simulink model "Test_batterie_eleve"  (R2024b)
settings: Solver=VariableStepAuto  StartTime=0.0  StopTime=288000  RelTol=1e-3
libraries: fl_lib x7, nesl_utility x6, ee_lib x4, simulink x2, batteryecm_lib x1, simulink_extras x1

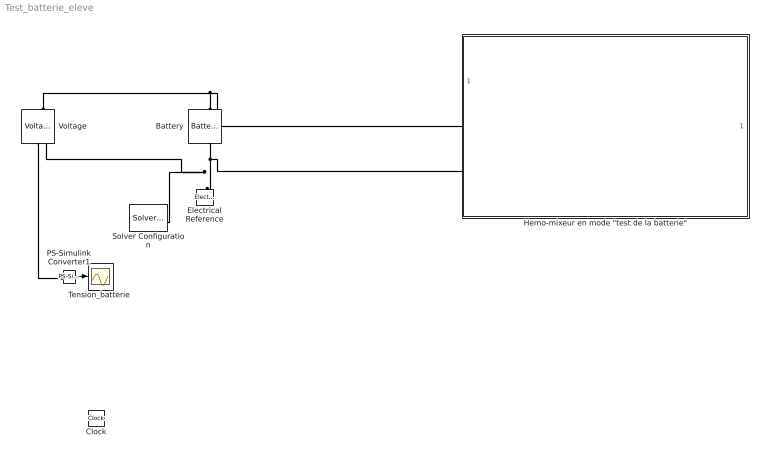
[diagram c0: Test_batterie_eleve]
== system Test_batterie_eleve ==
  Battery : batteryecm_lib/Battery  Vnom=9 V  prm_dir=simscape.enum.battery.prm_dir.disabled  R1_dis=2 Ohm  R1_ch=2 Ohm  R1=0.2 Ohm  prm_AH=2  AH=5 Ah  V1=10.8 V  AH1=0.76 Ah  prm_R2=1  R2=2000 Ohm  Tmeas=298.15 K  charge_measurement_port=simscape.enum.battery.enable.no  prm_dyn=1  Rp1=0.005 Ohm  tau1=30 s  Rp2=0.005 Ohm  tau2=30 s  Rp3=0.005 Ohm  tau3=30 s  Rp4=0.005 Ohm  tau4=30 s  Rp5=0.005 Ohm  tau5=30 s  prm_fade=1  N_fade=100  AH_fade=45 hr*A  R1_fade=2.02 Ohm  R1_ch_fade=2.02 Ohm  V1_fade=10.35 V  prm_age=simscape.enum.battery.prm_age.disabled  prm_age_OCV=simscape.enum.battery.prm_age_OCV.OCV  OCV_age=0.9  SOC_age=60  Tmeas_age=298.15 K  delta_time_age_vec=[0] d  temperature_age_vec=[273] K  OCV_scaling_age=2.2134e6  OCV_offset_age=1.632e6  temp_exp_age=0.515833569 V  t_exp_age=0.75  Vnom_T2=12 V  R1_T2=2.2 Ohm  R1_T2_dis=2.2 Ohm  R1_T2_ch=2.2 Ohm  V1_T2=11.4 V  R2_T2=2200 Ohm  Rp1_T2=0.005 Ohm  tau1_T2=30 s  Rp2_T2=0.005 Ohm  tau2_T2=30 s  Rp3_T2=0.005 Ohm  tau3_T2=30 s  Rp4_T2=0.005 Ohm  tau4_T2=30 s  Rp5_T2=0.005 Ohm  tau5_T2=30 s  Tmeas2=273.15 K  thermal_port=simscape.enum.thermaleffects.omit  thermal_mass=30000 J/K  i_specify=off  i_priority=None  i=0 A  i_nominal_specify=off  i_nominal_value=1  i_nominal_unit=A  v_specify=off  v_priority=None  v=14 V  v_nominal_specify=off  v_nominal_value=1  v_nominal_unit=V  charge_specify=on  charge_priority=High  charge=3.8 hr*A  charge_nominal_specify=off  charge_nominal_value=1  charge_nominal_unit=hr*A  num_cycles_specify=off  num_cycles_priority=High  num_cycles=0  num_cycles_nominal_specify=off  num_cycles_nominal_value=1  num_cycles_nominal_unit=1  temperature_specify=off  temperature_priority=High  temperature=298.15 K  temperature_nominal_specify=off  temperature_nominal_value=1  temperature_nominal_unit=K
  Electrical Reference : fl_lib/Electrical/Electrical Elements/Electrical Reference
  "Hemo-mixeur en mode \"test de la batterie\"" : Subsystem
  PS-Simulink Converter1 : nesl_utility/PS-Simulink Converter  PhysicalDomain=network_engine_domain  SubClassName=ps_output  LeftPortType=input  RightPortType=output  PseudoPeriodic=off  Frequencies=[]  VectorFormat=1-D array  Unit=inherit  AffineConversion=off
  Solver Configuration : nesl_utility/Solver Configuration  PhysicalDomain=network_engine_domain  SubClassName=solver  LeftPortType=input  RightPortType=generic  Tones=[]  Harmonics=[]  SimulateNoise=off  Profile=off  UseLocalSampling=off  EnableSwitchedLinearOptims=on  FrequencyDomain=off  UseCCode=off  RelTol=0.001  AbsTol=1e-06  MinStep=1e-09  ToWorkspace=off  RevertToSquareIcSolve=off  NumHomotopyIterations=100  PhasorMode=off  PhasorModeNumHarmonics=1  ConsistencySolver=NEWTON_FTOL  IndexReductionMethod=DerivativeReplacement  DoDC=off  ResidualTolerance=1e-09  ConsistencyTolSource=GLOBAL  ConsistencyAbsTol=0.001  ConsistencyRelTol=0.001  ConsistencyTolFactor=0.001  UseLocalSolver=off  LocalSolverChoice=NE_BACKWARD_EULER_ADVANCER  ResolveIndetEquations=on  FunctionEvalNumThread=1  LocalSolverSampleTime=0.001  DoFixedCost=off  MaxNonlinIter=3  MaxModeIter=2  ComputeImpulses=off  ImpulseIterations=2  LinearAlgebra=auto  LinearAlgebraNumThread=0  EquationFormulation=NE_TIME_EF  DelaysMemoryBudget=1024  AutomaticFiltering=on  FilteringTimeConstant=0.001  PartitionStorageMethod=AS_NEEDED  PartitionMemoryBudget=1024  PartitionMethod=ROBUST  MultibodyUseLocalSolver=off  MultibodyLocalSolverChoice=ODE1  MultibodyLocalSolverSampleTime=0.001
  "Tension_batterie " : Scope
  Voltage : fl_lib/Electrical/Electrical Sensors/Voltage Sensor
  Clock : Clock
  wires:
  PS-Simulink Converter1/1 -> "Tension_batterie "/1
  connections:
  Voltage/RConn1 -- PS-Simulink Converter1/LConn1
  Voltage/LConn1 -- "Hemo-mixeur en mode \"test de la batterie\""/LConn1 -- Battery/LConn1
  Battery/RConn1 -- Solver Configuration/RConn1 -- Voltage/RConn2 -- "Hemo-mixeur en mode \"test de la batterie\""/LConn2 -- Electrical Reference/LConn1

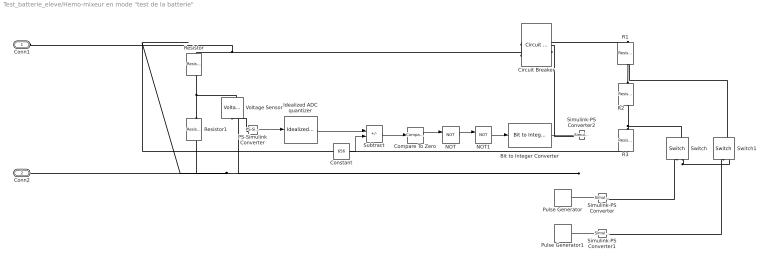
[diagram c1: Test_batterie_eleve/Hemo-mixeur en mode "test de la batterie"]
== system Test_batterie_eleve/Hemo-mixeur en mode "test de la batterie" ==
  Bit to Integer Converter : simulink/Logic and Bit Operations/Bit to Integer Converter  nbits=1  bitOrder=MSB first  signedOutputValues=Unsigned  outDtype=double  outDtypeSigned=Inherit via internal rule
  Circuit Breaker : ee_lib/Switches & Breakers/Circuit Breaker  R_closed=0.001 Ohm  G_open=1e-6 1/Ohm  threshold=0.5 V  breaker_behavior=ee.enum.switches.breakerBehavior.zeroCrossingDisable
  Compare To Zero : simulink/Logic and Bit Operations/Compare To Zero  relop=<=  OutDataTypeStr=boolean  ZeroCross=off
  Constant : Constant  Value=656
  Idealized ADC quantizer : simulink_extras/Additional Discrete/Idealized ADC quantizer  NumberOfConverterBits=10  Vmin=0  Vmax=5  OutputDataType=uint32  OutputNegativeValues=off
  NOT : Logic  Operator=NOT  IconShape=distinctive  AllPortsSameDT=off  OutDataTypeStr=boolean
  NOT1 : Logic  Operator=NOT  IconShape=distinctive  AllPortsSameDT=off
  PS-Simulink Converter : nesl_utility/PS-Simulink Converter  PhysicalDomain=network_engine_domain  SubClassName=ps_output  LeftPortType=input  RightPortType=output  PseudoPeriodic=off  Frequencies=[]  VectorFormat=inherit  Unit=inherit  AffineConversion=off
  Pulse Generator : DiscretePulseGenerator  PulseType=Time based  Period=120  PulseWidth=8.3  VectorParams1D=off
  Pulse Generator1 : DiscretePulseGenerator  PulseType=Time based  Period=120  PulseWidth=8.3  PhaseDelay=60  VectorParams1D=off
  R1 : ee_lib/Passive/Resistor  R=86 Ohm  enable_R_tol=1  R_tol=1  tol_distribution=1  nSigma=4  enable_operating_limits=0  operating_limit_action=2  power_rating=1 W  max_working_voltage=100 V  noise_mode=0  Tdevice=25 degC  sample_time=1e-3 s  repeatability=1  user_seed=0  auto_seed=3264415495  fault_action=simscape.enum.assert.action.none  t_fault=1 s  power_derating_T1=70 degC  power_derating_T2=155 degC  operating_temperature_range_vec=[-50, 150] degC  alpha=3.93e-3 1/K  Tmeas=25 degC  thermal_mass=100 J/K  temperature_specify=off  temperature_priority=High  temperature=298.15 K  temperature_nominal_specify=off  temperature_nominal_value=1  temperature_nominal_unit=K
  R2 : ee_lib/Passive/Resistor  R=14 Ohm  enable_R_tol=1  R_tol=1  tol_distribution=1  nSigma=4  enable_operating_limits=0  operating_limit_action=2  power_rating=1 W  max_working_voltage=100 V  noise_mode=0  Tdevice=25 degC  sample_time=1e-3 s  repeatability=1  user_seed=0  auto_seed=3467225173  fault_action=simscape.enum.assert.action.none  t_fault=1 s  power_derating_T1=70 degC  power_derating_T2=155 degC  operating_temperature_range_vec=[-50, 150] degC  alpha=3.93e-3 1/K  Tmeas=25 degC  thermal_mass=100 J/K  temperature_specify=off  temperature_priority=High  temperature=298.15 K  temperature_nominal_specify=off  temperature_nominal_value=1  temperature_nominal_unit=K
  R3 : ee_lib/Passive/Resistor  R=200 Ohm  enable_R_tol=1  R_tol=1  tol_distribution=1  nSigma=4  enable_operating_limits=0  operating_limit_action=2  power_rating=1 W  max_working_voltage=100 V  noise_mode=0  Tdevice=25 degC  sample_time=1e-3 s  repeatability=1  user_seed=0  auto_seed=4244480622  fault_action=simscape.enum.assert.action.none  t_fault=1 s  power_derating_T1=70 degC  power_derating_T2=155 degC  operating_temperature_range_vec=[-50, 150] degC  alpha=3.93e-3 1/K  Tmeas=25 degC  thermal_mass=100 J/K  temperature_specify=off  temperature_priority=High  temperature=298.15 K  temperature_nominal_specify=off  temperature_nominal_value=1  temperature_nominal_unit=K
  Resistor : fl_lib/Electrical/Electrical Elements/Resistor  R=23.7 kOhm  i_specify=off  i_priority=None  i=0 A  i_nominal_specify=off  i_nominal_value=1  i_nominal_unit=A  v_specify=off  v_priority=None  v=0 V  v_nominal_specify=off  v_nominal_value=1  v_nominal_unit=V
  Resistor1 : fl_lib/Electrical/Electrical Elements/Resistor  R=10 kOhm  i_specify=off  i_priority=None  i=0 A  i_nominal_specify=off  i_nominal_value=1  i_nominal_unit=A  v_specify=off  v_priority=None  v=0 V  v_nominal_specify=off  v_nominal_value=1  v_nominal_unit=V
  Simulink-PS Converter : nesl_utility/Simulink-PS Converter  PhysicalDomain=network_engine_domain  SubClassName=ps_input  LeftPortType=input  RightPortType=output  PseudoPeriodic=off  Frequencies=[]  NoiseDistribution=none  NoiseParameters=[]  Unit=1  AffineConversion=off  FilteringAndDerivatives=provide  SimscapeFilterOrder=1  InputFilterTimeConstant=0.001  UdotUserProvided=0
  Simulink-PS Converter1 : nesl_utility/Simulink-PS Converter  PhysicalDomain=network_engine_domain  SubClassName=ps_input  LeftPortType=input  RightPortType=output  PseudoPeriodic=off  Frequencies=[]  NoiseDistribution=none  NoiseParameters=[]  Unit=1  AffineConversion=off  FilteringAndDerivatives=provide  SimscapeFilterOrder=1  InputFilterTimeConstant=0.001  UdotUserProvided=0
  Simulink-PS Converter2 : nesl_utility/Simulink-PS Converter  PhysicalDomain=network_engine_domain  SubClassName=ps_input  LeftPortType=input  RightPortType=output  PseudoPeriodic=off  Frequencies=[]  NoiseDistribution=none  NoiseParameters=[]  Unit=1  AffineConversion=off  FilteringAndDerivatives=provide  SimscapeFilterOrder=1  InputFilterTimeConstant=0.001  UdotUserProvided=0
  Subtract : Sum  Inputs=+-
  Switch : fl_lib/Electrical/Electrical Elements/Switch  R_closed=0.01 Ohm  G_open=1e-8 1/Ohm  Threshold=0.5  i_specify=off  i_priority=None  i=0 A  i_nominal_specify=off  i_nominal_value=1  i_nominal_unit=A  v_specify=off  v_priority=None  v=0 V  v_nominal_specify=off  v_nominal_value=1  v_nominal_unit=V
  Switch1 : fl_lib/Electrical/Electrical Elements/Switch  R_closed=0.01 Ohm  G_open=1e-8 1/Ohm  Threshold=0.5  i_specify=off  i_priority=None  i=0 A  i_nominal_specify=off  i_nominal_value=1  i_nominal_unit=A  v_specify=off  v_priority=None  v=0 V  v_nominal_specify=off  v_nominal_value=1  v_nominal_unit=V
  Voltage Sensor : fl_lib/Electrical/Electrical Sensors/Voltage Sensor
  Conn1 : PMIOPort  Side=Left
  Conn2 : PMIOPort  Port=2  Side=Left
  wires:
  Pulse Generator/1 -> Simulink-PS Converter/1
  Pulse Generator1/1 -> Simulink-PS Converter1/1
  PS-Simulink Converter/1 -> Idealized ADC quantizer/1
  Constant/1 -> Subtract/2
  Idealized ADC quantizer/1 -> Subtract/1
  Subtract/1 -> Compare To Zero/1
  Compare To Zero/1 -> NOT/1
  NOT/1 -> NOT1/1
  NOT1/1 -> Bit to Integer Converter/1
  Bit to Integer Converter/1 -> Simulink-PS Converter2/1
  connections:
  R1/RConn1 -- Switch1/LConn1 -- R2/LConn1
  R3/LConn1 -- Switch/LConn1 -- R2/RConn1
  Switch/RConn2 -- Switch1/RConn2 -- Voltage Sensor/RConn2 -- Resistor1/RConn1 -- Conn2/RConn1 -- R3/RConn1
  Simulink-PS Converter/RConn1 -- Switch/RConn1
  Simulink-PS Converter1/RConn1 -- Switch1/RConn1
  Resistor1/LConn1 -- Voltage Sensor/LConn1 -- Resistor/RConn1
  PS-Simulink Converter/LConn1 -- Voltage Sensor/RConn1
  Circuit Breaker/LConn1 -- Simulink-PS Converter2/RConn1
  Circuit Breaker/LConn2 -- R1/LConn1
  Circuit Breaker/RConn1 -- Resistor/LConn1 -- Conn1/RConn1
